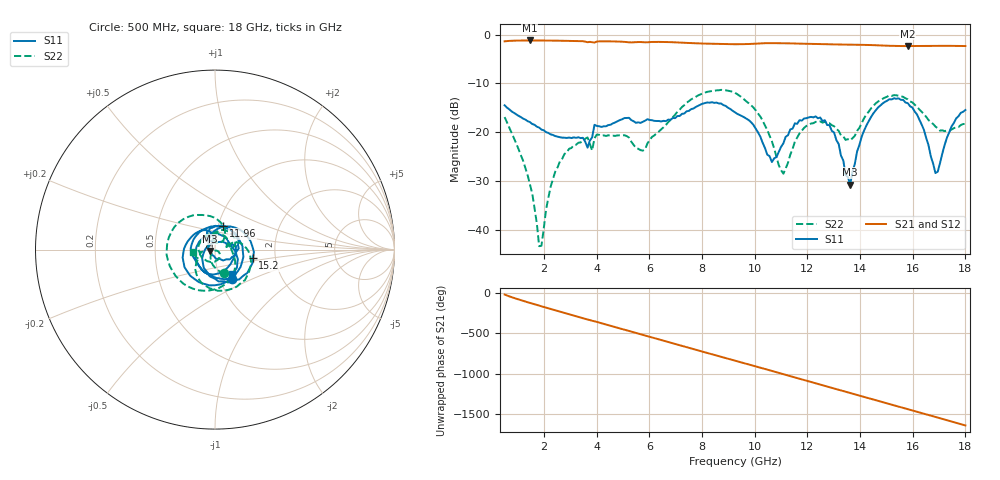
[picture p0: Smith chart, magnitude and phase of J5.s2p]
!Agilent Technologies,N5230C,MY49001096,A.09.42.15
!Agilent N5230C: A.09.42.15
!Date: Thursday, June 29, 2023 08:14:24
!Correction: S11(Full 2 Port(1,2))
!S21(Full 2 Port(1,2))
!S12(Full 2 Port(1,2))
!S22(Full 2 Port(1,2))
!S2P File: Measurements: S11, S21, S12, S22:
# Hz S  dB  R 50
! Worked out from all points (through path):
!   201 points, 500 MHz to 18 GHz, reference 50 ohm
!   highest |S21| = -1.22 dB at 1.462 GHz (marker M1); lowest = -2.4 dB at 15.81 GHz (marker M2)
!   group delay of S21, straight-line fit = 254 ps
!   lowest |S11| = -30.7 dB at 13.62 GHz (marker M3), VSWR 1.06, Z = 47.3 - j0.705 ohm
!   |S11| at or under -10 dB: start of sweep to end of sweep
!   |S22| runs from -43.3 to -11.3 dB; largest |S21 - S12| = 0.0013
!   S11 on the Smith chart (normalised r, x): 500 MHz: 1.14, -0.39; 11.96 GHz: 1.06, +0.28; 15.2 GHz: 1.53, -0.15; 18 GHz: 1.16, -0.33
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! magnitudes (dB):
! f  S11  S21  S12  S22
! 500 MHz  -14.5  -1.4  -1.4  -16.9
! 1.462 GHz  -17.9  -1.2  -1.2  -30.7
! 1.9 GHz  -19.5  -1.2  -1.2  -43.3
! 2.425 GHz  -20.8  -1.3  -1.3  -28.0
! 3.475 GHz  -21.2  -1.4  -1.4  -21.8
! 5.75 GHz  -17.9  -1.6  -1.6  -23.8
! 6.362 GHz  -17.7  -1.5  -1.5  -19.9
! 7.85 GHz  -14.6  -1.8  -1.8  -12.5
! 9.25 GHz  -15.9  -2.0  -2.0  -12.0
! 10.65 GHz  -26.1  -1.8  -1.8  -21.8
! 11.09 GHz  -22.3  -1.8  -1.8  -28.5
! 11.96 GHz  -17.1  -1.9  -1.9  -18.7
! 12.22 GHz  -17.0  -1.9  -1.9  -18.2
! 13.01 GHz  -20.1  -2.0  -2.0  -18.8
! 13.62 GHz  -30.7  -2.1  -2.1  -21.7
! 14.24 GHz  -18.7  -2.1  -2.1  -16.4
! 15.11 GHz  -13.3  -2.3  -2.3  -12.5
! 15.2 GHz  -13.3  -2.3  -2.3  -12.6
! 15.81 GHz  -14.1  -2.4  -2.4  -13.3
! 16.43 GHz  -19.5  -2.3  -2.3  -16.3
! 16.86 GHz  -28.4  -2.3  -2.3  -18.8
! 18 GHz  -15.5  -2.4  -2.4  -18.3
